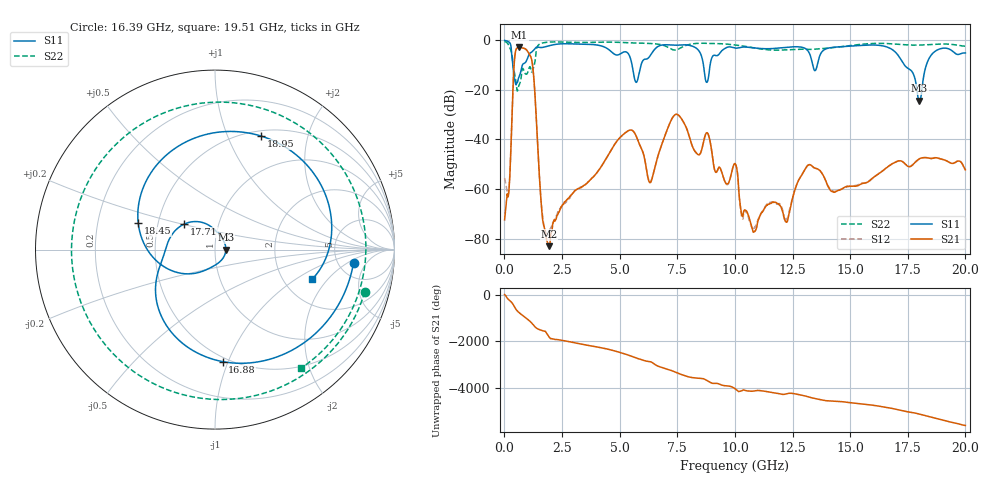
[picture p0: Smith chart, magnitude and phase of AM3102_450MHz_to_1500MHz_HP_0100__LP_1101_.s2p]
!Agilent Technologies,E8364B,MY43040894,A.07.50.67
!Agilent E8364B: A.07.50.67
!Date: Thursday, January 11, 2018 05:38:29
!Correction: S11(Full 2 Port(1,2))
!S21(Full 2 Port(1,2))
!S12(Full 2 Port(1,2))
!S22(Full 2 Port(1,2))
!S2P File: Measurements: S11, S21, S12, S22:
# Hz S  dB  R 50
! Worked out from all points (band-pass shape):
!   1601 points, 10 MHz to 20 GHz, reference 50 ohm
!   highest |S21| = -2.82 dB at 647.2 MHz (marker M1); lowest = -83.1 dB at 1.934 GHz (marker M2)
!   |S21| within 3 dB of the highest: 460.8 MHz to 1.098 GHz (637.2 MHz wide, 81.7 % of centre)
!   lowest |S11| = -24.4 dB at 18 GHz (marker M3), VSWR 1.13, Z = 56.4 - j0.0592 ohm
!   |S11| at or under -10 dB: 366.3 MHz to 779.9 MHz (413.6 MHz wide, 72.2 % of centre); 5.54 GHz to 5.927 GHz (387.1 MHz wide, 6.75 % of centre); 17.36 GHz to 18.3 GHz (949.4 MHz wide, 5.32 % of centre)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
!   |S22| runs from -20.4 to -0.5 dB; largest |S21 - S12| = 0.0024
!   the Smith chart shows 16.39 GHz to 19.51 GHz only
!   S11 on the Smith chart (normalised r, x): 16.39 GHz: 6.97, -2.53; 16.88 GHz: 0.47, -0.96; 17.71 GHz: 0.68, +0.20; 18.45 GHz: 0.39, +0.14; 18.95 GHz: 0.56, +1.33; 19.51 GHz: 2.88, -1.39
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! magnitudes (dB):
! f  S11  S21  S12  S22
! 10 MHz  -0.1  -72.4  -55.5  -0.5
! 184.9 MHz  -0.6  -61.9  -61.2  -2.0
! 447.3 MHz  -15.8  -7.0  -7.0  -13.6
! 647.2 MHz  -14.5  -2.8  -2.8  -17.9
! 1.197 GHz  -4.7  -8.4  -8.4  -12.7
! 1.634 GHz  -2.9  -69.9  -69.0  -1.1
! 1.934 GHz  -2.2  -83.1  -78.1  -0.7
! 3.346 GHz  -1.5  -59.2  -59.1  -0.9
! 6.682 GHz  -2.4  -46.1  -46.1  -1.6
! 7.481 GHz  -2.0  -29.9  -29.9  -3.8
! 10.01 GHz  -3.1  -49.7  -49.9  -1.9
! 10.84 GHz  -3.1  -77.2  -75.6  -3.1
! 13.34 GHz  -8.6  -50.7  -50.8  -3.7
! 16.39 GHz  -2.2  -52.9  -52.8  -1.2
! 16.68 GHz  -3.0  -50.7  -50.8  -1.3
! 16.88 GHz  -4.1  -49.6  -49.5  -1.5
! 17.71 GHz  -13.0  -50.2  -50.3  -1.9
! 18 GHz  -24.4  -47.8  -47.9  -1.9
! 18.45 GHz  -6.9  -47.6  -47.6  -1.7
! 18.95 GHz  -3.3  -47.9  -47.9  -1.5
! 19.51 GHz  -4.9  -49.5  -49.4  -1.8
! 20 GHz  -5.1  -52.2  -52.5  -2.4
